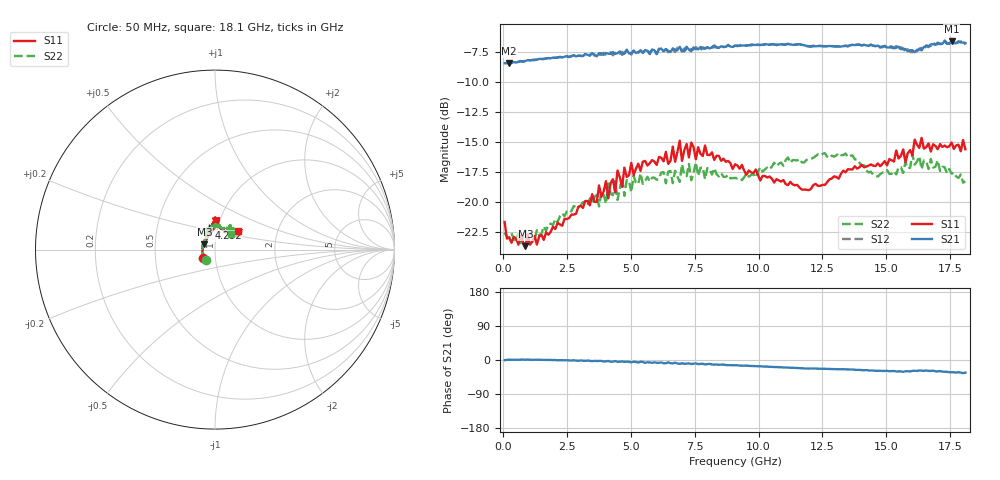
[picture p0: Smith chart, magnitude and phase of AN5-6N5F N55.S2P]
! Network Analyzer HP8720D.06.14 Serial No. US36140669
!  6 Jul 2005  08:12:51
! Frequency  S11  S21  S12  S22
# HZ  S  DB R 50
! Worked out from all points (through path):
!   201 points, 50 MHz to 18.1 GHz, reference 50 ohm
!   highest |S21| = -6.59 dB at 17.56 GHz (marker M1); lowest = -8.4 dB at 230.5 MHz (marker M2)
!   group delay of S21, straight-line fit = 5.85 ps
!   lowest |S11| = -23.7 dB at 862.2 MHz (marker M3), VSWR 1.14, Z = 44.4 + j2.56 ohm
!   |S11| at or under -10 dB: start of sweep to end of sweep
!   |S22| runs from -23.5 to -15.9 dB; largest |S21 - S12| = 0.018
!   S11 on the Smith chart (normalised r, x): 50 MHz: 0.87, -0.09; 4.292 GHz: 0.91, +0.22; 18.1 GHz: 1.27, +0.27
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5e7  -21.67 -143.7  -8.43 -0.4  -8.42 -0.2  -22.55 -129.8
2.305e8  -22.98 -174.1  -8.45 1.0  -8.46 0.8  -22.98 -176.5
8.6225e8  -23.68 154.0  -8.25 0.8  -8.23 0.9  -22.38 160.4
9.525e8  -22.69 154.1  -8.17 1.1  -8.23 1.1  -23.50 155.3
3.1185e9  -20.50 111.8  -7.82 -1.6  -7.84 -2.0  -20.01 121.0
4.021e9  -18.27 103.3  -7.57 -3.5  -7.71 -2.7  -20.14 111.9
4.11125e9  -19.69 101.7  -7.64 -2.5  -7.62 -4.0  -18.46 110.7
4.29175e9  -18.10 105.2  -7.49 -4.2  -7.77 -4.2  -19.44 104.4
6.09675e9  -16.25 89.8  -7.26 -7.4  -7.21 -7.3  -18.06 97.8
6.7285e9  -16.64 92.8  -7.30 -6.9  -7.50 -8.0  -17.39 90.6
6.909e9  -14.89 89.8  -7.07 -10.2  -7.25 -8.8  -18.33 87.7
6.99925e9  -16.58 89.1  -7.39 -8.6  -7.45 -10.3  -16.84 88.9
7.36025e9  -15.04 82.3  -7.44 -10.5  -7.24 -9.3  -18.18 91.9
7.54075e9  -16.44 83.0  -7.23 -8.9  -7.09 -11.1  -16.69 90.4
7.90175e9  -15.30 86.8  -7.22 -11.7  -7.17 -10.4  -18.09 84.2
9.075e9  -16.86 85.7  -6.97 -13.8  -6.95 -13.9  -17.99 73.1
1.21435e10  -18.59 59.5  -7.00 -22.3  -6.96 -22.5  -16.32 59.2
1.512175e10  -16.42 31.1  -7.12 -29.6  -6.97 -29.3  -17.66 52.5
1.602425e10  -16.10 36.2  -7.35 -28.6  -7.52 -30.4  -16.02 49.5
1.61145e10  -14.80 34.9  -7.51 -28.5  -7.24 -28.6  -16.89 51.4
1.75585e10  -15.04 40.0  -6.59 -32.3  -6.60 -32.3  -17.64 49.6
1.81e10  -15.61 38.2  -6.74 -33.4  -6.88 -33.9  -18.28 44.2
